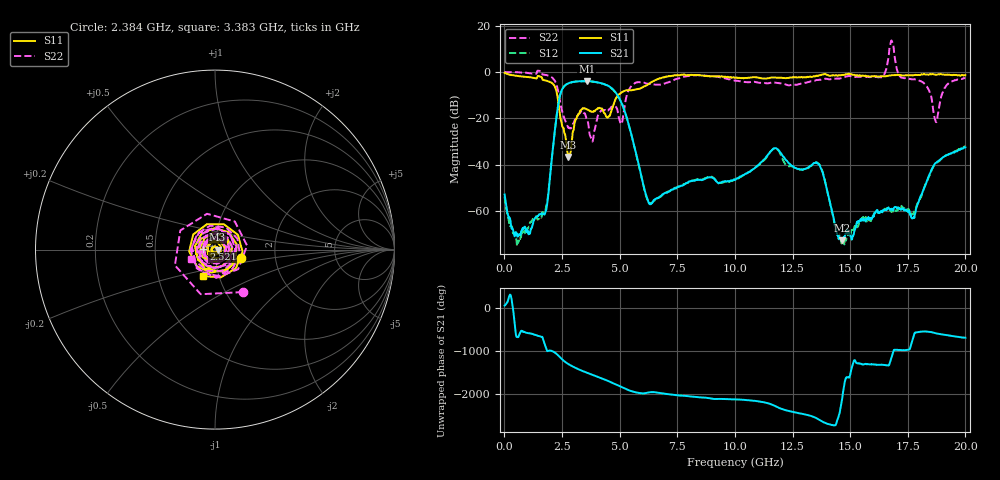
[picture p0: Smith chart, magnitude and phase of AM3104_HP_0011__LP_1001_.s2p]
!Created with skrf (http://scikit-rf.org).
# Hz S RI R 50.0
!freq ReS11 ImS11 ReS21 ImS21 ReS12 ImS12 ReS22 ImS22
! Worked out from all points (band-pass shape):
!   1601 points, 10 MHz to 20 GHz, reference 50 ohm
!   highest |S21| = -3.95 dB at 3.571 GHz (marker M1); lowest = -72.7 dB at 14.64 GHz (marker M2)
!   |S21| within 3 dB of the highest: 2.536 GHz to 4.649 GHz (2.113 GHz wide, 58.8 % of centre)
!   lowest |S11| = -36.7 dB at 2.771 GHz (marker M3), VSWR 1.03, Z = 51.5 + j0.053 ohm
!   |S11| at or under -10 dB: 2.293 GHz to 4.94 GHz (2.647 GHz wide, 73.2 % of centre)
!   |S22| runs from -30.0 to 13.6 dB; largest |S21 - S12| = 0.049
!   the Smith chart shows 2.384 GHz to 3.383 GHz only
!   S11 on the Smith chart (normalised r, x): 2.384 GHz: 1.33, -0.12; 2.521 GHz: 0.88, +0.01; 3.383 GHz: 0.84, -0.26
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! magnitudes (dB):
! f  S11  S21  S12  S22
! 10 MHz  -0.4  -52.9  -53.8  0.0
! 597.2 MHz  -1.8  -70.8  -73.7  -0.1
! 1.747 GHz  -3.6  -61.5  -60.6  -1.2
! 2.384 GHz  -16.4  -11.5  -11.5  -11.0
! 2.521 GHz  -23.8  -7.2  -7.2  -17.7
! 2.771 GHz  -36.7  -4.9  -4.9  -24.1
! 3.346 GHz  -16.2  -4.0  -4.1  -16.8
! 3.383 GHz  -15.8  -4.0  -4.1  -16.9
! 3.571 GHz  -16.1  -3.9  -4.0  -20.2
! 3.783 GHz  -17.1  -4.1  -4.1  -29.1
! 4.908 GHz  -10.4  -10.0  -10.1  -16.5
! 6.182 GHz  -5.7  -54.2  -54.7  -5.0
! 6.682 GHz  -3.0  -54.5  -54.3  -5.5
! 10.01 GHz  -2.5  -46.7  -46.5  -3.7
! 11.72 GHz  -2.4  -33.0  -33.1  -4.6
! 13.34 GHz  -2.1  -40.2  -40.2  -4.0
! 13.75 GHz  -1.3  -42.1  -41.7  -3.2
! 14.64 GHz  -1.3  -72.7  -73.6  -2.6
! 16.68 GHz  -1.6  -59.0  -59.4  7.2
! 17.74 GHz  -1.4  -62.8  -61.5  -3.2
! 18.71 GHz  -1.2  -39.3  -39.5  -21.4
! 20 GHz  -1.4  -32.6  -32.1  -2.6
